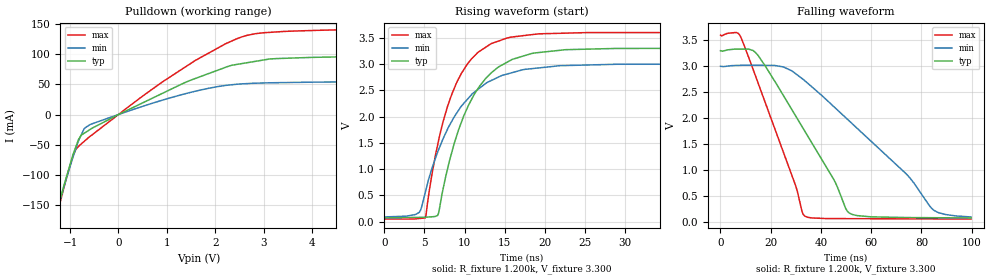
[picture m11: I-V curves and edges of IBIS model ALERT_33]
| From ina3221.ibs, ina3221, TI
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|   ALERT Open_drain Model
[Model]   ALERT_33
Model_type   Open_drain
Polarity   Non-Inverting
Vmeas = 1.65
Vref = 1.65
Cref = 2pF
Rref = 1200
|   typ   min   max
|   (nom PVT)   (Fast PVT)   (slow PVT)
|   ON state : BUFFER OUTPUT TURNED HIGH
C_comp   1.248E-12   1.029E-12   1.500E-12
|   OFF state: BUFFER OUTPUT TURNED LOW
|C_comp   9.596E-13   8.552E-13   1.154E-12
| Where   nom PVT is  Nominal Process, 3.3V, 25C
|   Fast PVT is Strong Process, 3.6V, -40C
|   Slow PVT is Weak Process, 3.0V, 85C
|C_comp - from L-C Tank method, L = 1nH, peak frequency
[Voltage Range]   3.3   3   3.6
|Ambient Temperature Range   27   85   -40
[Temperature Range]   30   88   -40
[Pullup Reference]   3.3   3   3.6
[Pulldown Reference]   0   0   0
[Power Clamp Reference]   3.3   3   3.6
[GND Clamp Reference]   0   0   0
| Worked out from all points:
|   slope of the pulldown table from 0 to 0.495 V, typ, clamps not added: 25.9 ohm
|   falling waveform, R_fixture 1.200k, V_fixture 3.300: 20-80 % time 23.8ns typ, 37.3ns min, 16.1ns max; typ from 3.3 V to 0.07 V
|   rising waveform, R_fixture 1.200k, V_fixture 3.300: 20-80 % time 4.81ns typ, 5.57ns min, 4.1ns max; typ from 0.07 V to 3.3 V
[Pulldown]
|   Voltage   I(typ)   I(min)   I(max)
-3.3V     -810.3mA   -771mA     -893.9mA
-1.368V   -188.1mA   -187.1mA   -195.9mA
-1.15V    -124.1mA   -125.6mA   -128.1mA
-923.2mV  -62.65mA   -66.61mA   -64.57mA
-827.2mV  -41.47mA   -43.82mA   -52.85mA
-692.7mV  -30.18mA   -22.11mA   -43.37mA
902.6mV   34.84mA    23.65mA    53.68mA
1.59V     59.73mA    38.59mA    89.63mA
2.439V    82.89mA    50.12mA    125.3mA
2.833V    88.13mA    51.87mA    133.9mA
3.424V    93.1mA     52.91mA    137.7mA
6.59V     97.96mA    55.35mA    144.2mA
[Ramp]
R_load = 1200
|   typ   min   max
dV/dt_r   1.93822/4.8008e-009   1.71821/5.57595e-009   2.13117/4.09188e-009
dV/dt_f   1.93819/2.37849e-008   1.7179/3.73599e-008   2.13117/1.6065e-008
[Falling Waveform]
R_fixture = 1.200k
V_fixture = 3.300
V_fixture_min = 3.000
V_fixture_max = 3.600
C_fixture = 0.000
|  time   V(typ)   V(min)   V(max)
0s        3.3V       3V         3.6V
8.157ns   3.33V      3.018V     3.554V
14.77ns   3.219V     3.018V     2.702V
25.03ns   2.435V     2.986V     1.341V
33.51ns   1.75V      2.723V     107.4mV
45.17ns   806.9mV    2.217V     56.93mV
51.47ns   159.3mV    1.934V     55.9mV
74.26ns   76.91mV    905.1mV    52.2mV
84.81ns   73.92mV    222.4mV    50.49mV
99.76ns   69.69mV    88.18mV    48.06mV
[Rising Waveform]
R_fixture = 1.200k
V_fixture = 3.300
V_fixture_min = 3.000
V_fixture_max = 3.600
C_fixture = 0.000
|  time   V(typ)   V(min)   V(max)
0s        69.64mV    88.18mV    48.05mV
4.351ns   79.88mV    172.8mV    58.26mV
5.113ns   82.39mV    553.2mV    69.64mV
6.655ns   118.4mV    1.323V     1.462V
8.421ns   1.322V     1.913V     2.427V
10.46ns   2.204V     2.345V     3.019V
12.69ns   2.733V     2.636V     3.324V
15.39ns   3.041V     2.812V     3.498V
28.94ns   3.296V     2.995V     3.597V
99.76ns   3.3V       3V         3.6V
